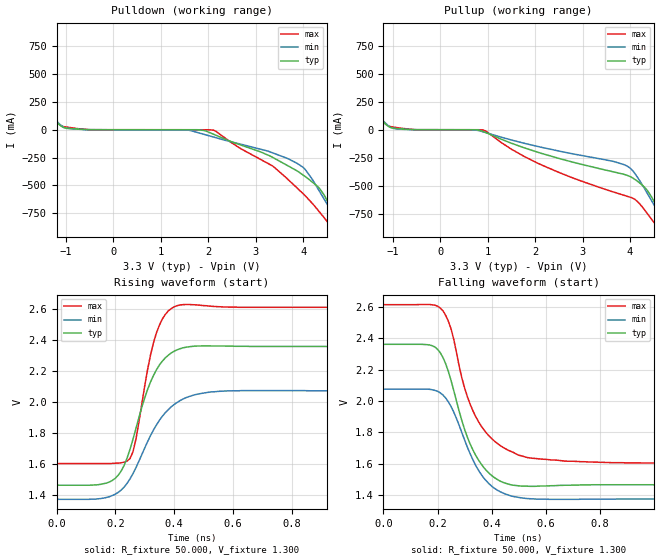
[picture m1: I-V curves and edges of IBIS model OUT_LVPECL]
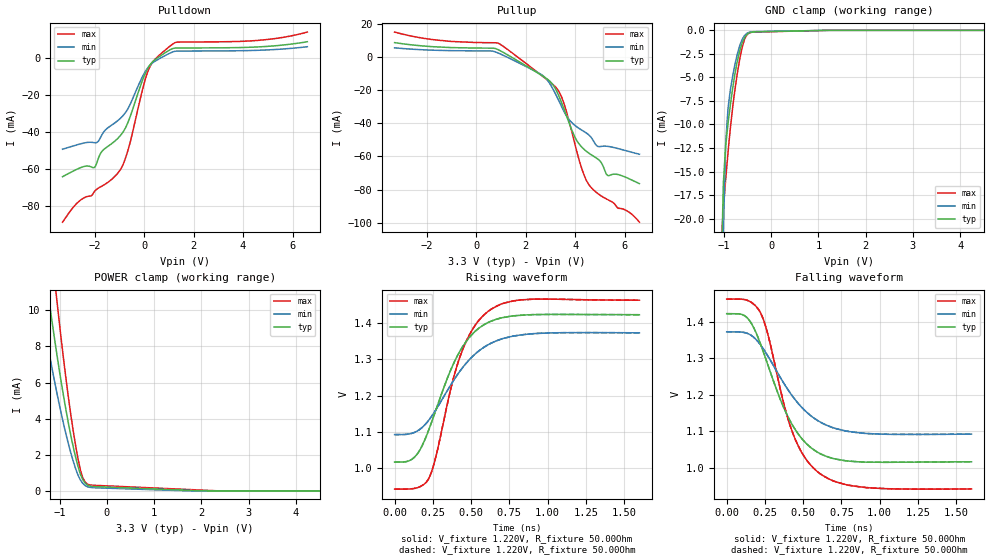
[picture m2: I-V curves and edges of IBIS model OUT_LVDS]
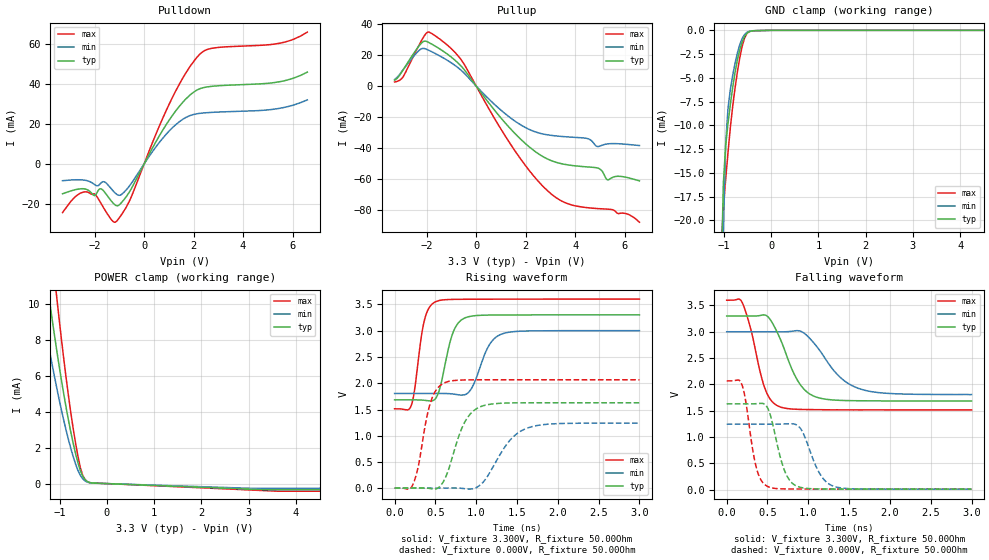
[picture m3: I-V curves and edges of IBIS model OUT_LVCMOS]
| Texas Instruments Incorporated
| Low-Noise Two-Channel 100-Mhz Clock Generator
| Marketing part#   Voltage Range   Package-type   #pins/pkg drawing
| CDCM9102   3.0V - 3.6V   QFN   32-pin
[IBIS ver]   4.0
[File name]   cdcm9102.ibs
[File Rev]   1.0
[Date]   02/xx/2012
[Source]   Texas Instruments Incorporated.
   Analog-eLab, HPA
   12500 TI Blvd
   Dallas, TX -75243
   For Support e-mail: elab_scm_ibis@list.ti.com
[Notes]   Revision History
   Rev 1.0: 02/xx/2012
   - Initial version of the model
   - Model based on simulations
[Disclaimer] This model is designed as an aid for customers of Texas Instruments.
 TI and its licensors and suppliers make no warranties, either expressed
 or implied, with respect to this  model, including the warranties of
 merchantability or fitness for a particular purpose.
 The model is provided solely on an "as is" basis. The entire risk as to
 its quality and performance is with the customer.
[Copyright] (C)Copyright 2012 Texas Instruments Incorporated.
   All rights reserved.
|   Component CDCM61001RHB
[Component]   CDCM9102
[Manufacturer]  Texas Instruments Incorporated
[Package]   |32-pin QFN RHB package + 1 mount pad
|   typ   min   max
R_pkg   0.0803   0.0465   0.1059
L_pkg   1.2961nH   0.9741nH   1.5599nH
C_pkg   0.1651pF   0.1340pF   0.2122pF
[Pin] signal_name  model_name   R_pin   L_pin   C_pin
1   VDD2   POWER   0.00347   0.14167nH   1.00649pF
2   OUT1N   OUT   0.10591   1.55991nH   0.16987pF
3   OUT1P   OUT   0.09554   1.38887nH   0.1537pF
4   VDD1   POWER   0.04649   0.97408nH   0.19897pF
5   OUT0N   OUT   0.0911   1.31619nH   0.14955pF
6   OUT0P   OUT   0.09304   1.34796nH   0.15105pF
7   OE   INPUT   0.09755   1.42251nH   0.15426pF
8   NC   NC   0.00035   0.05145nH   0.04372pF
9   VDD3   POWER   0.05784   1.4044nH   0.19557pF
10   OS1   INPUT   0.10035   1.46771nH   0.16304pF
11   OS0   INPUT   0.0874   1.25397nH   0.14393pF
12   RESETB   INPUT   0.07979   1.12929nH   0.13396pF
13   NC   NC   0.07954   1.12339nH   0.13334pF
14   GND   GND   0.08671   1.23786nH   0.13819pF
15   NC   NC   0.00035   0.04801nH   0.05605pF
16   VDD4   POWER   0.05695   1.35534nH   0.18238pF
17   REGCAP2   NC   0.1063   1.56176nH   0.15246pF
18   VDD5   POWER   0.05405   1.20242nH   0.21216pF
19   REGCAP1   NC   0.09847   1.42827nH   0.15881pF
20   VDD6   POWER   0.04904   1.04789nH   0.20348pF
21   XIN   NC   0.09225   1.32579nH   0.14835pF
22   GND   GND   0.09116   1.30806nH   0.14707pF
23   OSCOUT   OSC_OUT_25M   0.0919   1.32091nH   0.14396pF
24   NC   NC   0.00035   0.05145nH   0.04372pF
25   NC   NC   0.00035   0.05146nH   0.04372pF
26   NC   NC   0.00035   0.04801nH   0.05605pF
27   NC   NC   0.00035   0.04727nH   0.05608pF
28   NC   NC   0.00035   0.04709nH   0.05608pF
29   NC   NC   0.00035   0.04709nH   0.05608pF
30   NC   NC   0.00035   0.04726nH   0.05609pF
31   NC   NC   0.00035   0.04801nH   0.05605pF
32   NC   NC   0.00035   0.05145nH   0.04372pF
[Diff_Pin]  inv_pin  vdiff   tdelay_typ  tdelay_min  tdelay_max
| Driver Pins   |  Rload = 50 OHM to VCC-2 termination
|   Vdiff_lvpecl = 0.915V and Vdiff_lvds=0.350V
3   2   NA   0ns   0ns   0ns
6   5   NA   0ns   0ns   0ns
[Model Selector]   OUT
OUT_LVCMOS   LVCMOS OUTPUT
OUT_LVDS   LVDS   OUTPUT
OUT_LVPECL   LVPECL OUTPUT
| Models and submodels in the file (5): OUT_LVPECL (Output_ECL), OUT_LVDS (3-state), OUT_LVCMOS (3-state), OSC_OUT_25M (Output), INPUT (Input)
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|   OUT_LVPECL valid upto clock speed of 625MHz
[Model]   OUT_LVPECL
Model_type   Output_ECL
Cref = 0.0pF   |Timing specification test load capacitance value
Rref = 50.00Ohm
| variable   typ   min   max
|   Nominal PVT   Strong PVT   Weak PVT
C_comp   1.1664pF   1.1619pF   1.1764pF
[Model Spec]
Vref   1.3V   1.0V   1.6V
Vmeas   1.3V   1.0V   1.6V
[pullup reference]   3.3V   3.0V   3.6V
[pulldown reference]   3.3V   3.0V   3.6V
[GND clamp reference]   0V   0V   0V
| Junction Temperature (Ambient temp is 25C typ, 85C min,  -40C max)
[Temperature Range]   40.0   100.0   -40.0
[Voltage range]   3.3V   3.0V   3.6V
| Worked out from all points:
|   falling waveform, R_fixture 50.000, V_fixture 1.300: 20-80 % time 103ps typ, 110ps min, 118ps max; typ from 2.36 V to 1.47 V
|   rising waveform, R_fixture 50.000, V_fixture 1.300: 20-80 % time 91.4ps typ, 118ps min, 59.9ps max; typ from 1.47 V to 2.36 V
[Pulldown]
|   Voltage   I(typ)   I(min)   I(max)
-3.3V     1.332A     1.268A     1.424A
-2.68V    935.4mA    899.2mA    1.004A
-1.288V   115mA      119.3mA    116.2mA
-1.042V   18.84mA    20.53mA    27.56mA
1.586V    -109.5uA   -4.153mA   -17.03uA
2.111V    -40.58mA   -65.67mA   -4.131mA
3.352V    -247mA     -206.9mA   -324.1mA
3.992V    -405.1mA   -335.5mA   -571.5mA
4.342V    -525.1mA   -551.5mA   -737.5mA
4.689V    -781.1mA   -805.6mA   -932mA
4.89V     -953.1mA   -957.8mA   -1.114A
6.6V      -2.418A    -2.277A    -2.862A
[Pullup]
|   Voltage   I(typ)   I(min)   I(max)
-3.3V     1.332A     1.269A     1.435A
-2.63V    904.6mA    868.5mA    966.5mA
-1.29V    115.3mA    120.4mA    117.6mA
-1.067V   23.18mA    26.86mA    29.91mA
918mV     -17.48mA   -20.67mA   -4.542mA
2.059V    -201.7mA   -150.1mA   -300mA
3.672V    -378.5mA   -285.8mA   -559.7mA
4.02V     -422.7mA   -350mA     -605.8mA
4.317V    -519.2mA   -535mA     -722.3mA
4.665V    -763.2mA   -788.8mA   -915mA
4.838V    -904.1mA   -917.4mA   -1.054A
6.6V      -2.409A    -2.271A    -2.848A
[Ramp]
R_load = 50
|   typ   min   max
dV/dt_r   0.557474/9.12219e-11   0.420554/1.18318e-10   0.605849/5.99991e-11
dV/dt_f   0.557443/1.02721e-10   0.420514/1.10073e-10   0.605859/1.1832e-10
[Falling Waveform]
R_fixture = 50.000
V_fixture = 1.300
V_fixture_min = 1.000
V_fixture_max = 1.600
C_fixture = 0.000
|  time   V(typ)   V(min)   V(max)
0s        2.361V     2.075V     2.614V
170ps     2.357V     2.074V     2.615V
220ps     2.276V     2.037V     2.574V
250ps     2.128V     1.963V     2.457V
300ps     1.816V     1.749V     2.08V
340ps     1.654V     1.59V      1.902V
410ps     1.51V      1.442V     1.743V
500ps     1.458V     1.384V     NA
840ps     1.465V     1.373V     1.606V
1.7ns     1.465V     1.374V     1.605V
[Rising Waveform]
R_fixture = 50.000
V_fixture = 1.300
V_fixture_min = 1.000
V_fixture_max = 1.600
C_fixture = 0.000
|  time   V(typ)   V(min)   V(max)
0s        1.465V     1.374V     1.605V
180ps     1.486V     1.391V     1.605V
220ps     1.557V     1.434V     1.61V
250ps     1.696V     1.506V     1.637V
270ps     1.83V      1.577V     1.76V
310ps     2.084V     1.747V     2.213V
340ps     2.21V      1.854V     2.449V
410ps     2.339V     1.999V     2.624V
580ps     2.363V     2.074V     2.616V
1.7ns     2.361V     2.075V     2.614V
|   OUT_LVDS  valid upto clock speed of 625MHz
[Model]   OUT_LVDS
Model_type   3-state
Cref = 0.0pF   |Timing specification test load capacitance value
Rref = 50.00Ohm
| variable   typ   min   max
|   Nominal PVT   Strong PVT   Weak PVT
C_comp   1.1664pF   1.1619pF   1.1764pF
[Model Spec]
Vref   1.25V   1.15V   1.375V
Vmeas   1.25V   1.15V   1.375V
| Junction Temperature (Ambient temp is 25C typ, 85C min,  -40C max)
[Temperature Range]   40.0   100.0   -40.0
[Voltage range]   3.3V   3.0V   3.6V
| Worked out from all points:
|   slope of the pulldown table from 0 to 0.495 V, typ, clamps not added: 52.5 ohm
|   slope of the pullup table from 0 to 0.495 V, typ, clamps not added: 10.8 kohm
|   GND clamp passes 1 mA (typ) near -0.58 V on its own axis
|   POWER clamp passes 1 mA (typ) near -0.57 V on its own axis
|   falling waveform, V_fixture 1.220V, R_fixture 50.00Ohm: 20-80 % time 240ps typ, 280ps min, 211ps max; typ from 1.42 V to 1.02 V
|   rising waveform, V_fixture 1.220V, R_fixture 50.00Ohm: 20-80 % time 239ps typ, 282ps min, 200ps max; typ from 1.02 V to 1.42 V
|   rising waveform, V_fixture 1.220V, R_fixture 50.00Ohm: 20-80 % time 239ps typ, 282ps min, 200ps max; typ from 1.02 V to 1.42 V
|   falling waveform, V_fixture 1.220V, R_fixture 50.00Ohm: 20-80 % time 240ps typ, 280ps min, 211ps max; typ from 1.42 V to 1.02 V
[Pulldown]
|   Voltage   I(typ)   I(min)   I(max)
-3.3V     -64.32mA   -49.44mA   -88.92mA
-2.703V   -60.19mA   -47.03mA   -78.49mA
-2.007V   -59.31mA   -45.92mA   -72.26mA
-1.708V   -50.67mA   -41.67mA   -69.4mA
-961.8mV  -42.07mA   -32.76mA   -60.51mA
-613.6mV  -33.57mA   -26.49mA   -48.17mA
-66.33mV  -12.2mA    -10.21mA   -17.29mA
182.4mV   -4.943mA   -4.832mA   -6.331mA
431.2mV   -1.132mA   -1.934mA   -901.9uA
1.078V    4.53mA     2.728mA    6.643mA
4.909V    6.12mA     4.227mA    9.792mA
6.6V      8.704mA    6.006mA    13.92mA
[GND Clamp]
|   Voltage   I(typ)   I(min)   I(max)
-3.3V     -4.022A    -3.907A    -4.266A
-1.061V   -27.23mA   -43.89mA   -23.06mA
-1.012V   -16.24mA   -21.24mA   -18.95mA
-961.8mV  -12.25mA   -11.96mA   -15.82mA
-912.1mV  -9.874mA   -8.274mA   -12.94mA
-862.3mV  -7.89mA    -6.288mA   -10.34mA
-762.8mV  -4.522mA   -3.552mA   -6.176mA
-663.3mV  -2.151mA   -1.601mA   -3.015mA
-563.8mV  -779.3uA   -554.1uA   -972.9uA
-464.3mV  -264.9uA   -209.2uA   -276uA
1.227V    0A         -449.7nA   0A
6.6V      0A         0A         0A
[Pullup]
|   Voltage   I(typ)   I(min)   I(max)
-3.3V     8.704mA    5.566mA    15.07mA
878.9mV   4.518mA    2.501mA    8.413mA
2.521V    -9.902mA   -9.588mA   -9.69mA
3.068V    -16.07mA   -18.35mA   -16.17mA
3.416V    -26.18mA   -28.72mA   -22.91mA
4.013V    -48.96mA   -41.51mA   -53.82mA
4.312V    -55.01mA   -44.53mA   -69.18mA
4.56V     -58.06mA   -47.08mA   -77.11mA
4.909V    -61.49mA   -53.91mA   -82.32mA
5.307V    -71.46mA   -53.89mA   -85.99mA
5.754V    -71.01mA   -55.33mA   -91.31mA
6.6V      -76.42mA   -58.67mA   -99.7mA
[POWER Clamp]
|   Voltage   I(typ)   I(min)   I(max)
-3.3V     434.9mA    385mA      510.3mA
-1.459V   15.25mA    11.2mA     21.25mA
-1.41V    14.21mA    10.41mA    19.82mA
-1.26V    11.23mA    8.169mA    15.68mA
-1.211V   10.27mA    7.457mA    14.36mA
-1.061V   7.576mA    5.441mA    10.58mA
-862.3mV  4.403mA    3.086mA    6.102mA
-663.3mV  1.864mA    1.229mA    2.504mA
-514.1mV  630uA      424.6uA    736.8uA
-414.6mV  324.6uA    230.2uA    378.2uA
2.371V    0A         0A         2.594uA
6.6V      0A         0A         0A
[Ramp]
R_load = 50.00Ohm
|   typ   min   max
dV/dt_r   243.237mV/238.776ps 168.023mV/281.936ps 311.885mV/199.972ps
dV/dt_f   243.237mV/239.793ps 168.023mV/279.558ps 311.885mV/211.102ps
[Falling Waveform]
V_fixture = 1.220V
V_fixture_min = 1.232V
V_fixture_max = 1.200V
R_fixture = 50.00Ohm
|   Time   V(typ)   V(min)   V(max)
0s        1.422V     1.373V     1.462V
130ps     1.413V     1.369V     1.46V
220ps     1.34V      1.338V     1.425V
266ps     1.286V     1.308V     1.371V
372ps     1.166V     1.233V     1.178V
428ps     1.119V     1.198V     1.1V
503ps     1.074V     1.16V      1.034V
603ps     1.041V     1.128V     986.5mV
897ps     1.016V     1.095V     946.9mV
1.6ns     1.017V     1.092V     942.4mV
[Rising Waveform]
V_fixture = 1.220V
V_fixture_min = 1.232V
V_fixture_max = 1.200V
R_fixture = 50.00Ohm
|   Time   V(typ)   V(min)   V(max)
0s        1.017V     1.092V     942.4mV
128ps     1.03V      1.098V     944.3mV
223ps     1.105V     1.132V     971.5mV
265ps     1.154V     1.158V     1.024V
370ps     1.274V     1.231V     1.223V
429ps     1.324V     1.268V     1.309V
508ps     1.369V     1.307V     1.381V
610ps     1.401V     1.339V     1.431V
826ps     1.421V     1.367V     1.463V
1.6ns     1.422V     1.373V     1.462V
[Rising Waveform]
V_fixture = 1.220V
V_fixture_min = 1.232V
V_fixture_max = 1.200V
R_fixture = 50.00Ohm
|   Time   V(typ)   V(min)   V(max)
0s        1.017V     1.092V     942.4mV
128ps     1.03V      1.098V     944.3mV
223ps     1.105V     1.132V     971.5mV
265ps     1.154V     1.158V     1.024V
370ps     1.274V     1.231V     1.223V
429ps     1.324V     1.268V     1.309V
508ps     1.369V     1.307V     1.381V
610ps     1.401V     1.339V     1.431V
826ps     1.421V     1.367V     1.463V
1.6ns     1.422V     1.373V     1.462V
[Falling Waveform]
V_fixture = 1.220V
V_fixture_min = 1.232V
V_fixture_max = 1.200V
R_fixture = 50.00Ohm
|   Time   V(typ)   V(min)   V(max)
0s        1.422V     1.373V     1.462V
130ps     1.413V     1.369V     1.46V
220ps     1.34V      1.338V     1.425V
266ps     1.286V     1.308V     1.371V
372ps     1.166V     1.233V     1.178V
428ps     1.119V     1.198V     1.1V
503ps     1.074V     1.16V      1.034V
603ps     1.041V     1.128V     986.5mV
897ps     1.016V     1.095V     946.9mV
1.6ns     1.017V     1.092V     942.4mV
|   OUT_LVCMOS valid upto clock speed of 125MHz
[Model]   OUT_LVCMOS
Model_type   3-state
Cref = 5pF   |Timing specification test load capacitance value
Rref = 22Ohm
| variable   typ   min   max
|   Nominal PVT   Strong PVT   Weak PVT
C_comp   1.1795pF   1.1753pF   1.1905pF
[Model Spec]
|Timing spec test load voltage corners 0.45*VCC
Vmeas   3.3V   3.0V   3.6V
Vref   3.3V   3.0V   3.6V
| Junction Temperature (Ambient temp is 15C typ, 85C min,  -40C max)
[Temperature Range]   40.0   100.0   -40.0
[Voltage range]   3.3V   3.0V   3.6V
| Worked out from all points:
|   slope of the pulldown table from 0 to 0.495 V, typ, clamps not added: 43.1 ohm
|   slope of the pullup table from 0 to 0.495 V, typ, clamps not added: 46.8 ohm
|   GND clamp passes 1 mA (typ) near -0.59 V on its own axis
|   POWER clamp passes 1 mA (typ) near -0.60 V on its own axis
|   falling waveform, V_fixture 3.300V, R_fixture 50.00Ohm: 20-80 % time 273ps typ, 381ps min, 195ps max; typ from 3.3 V to 1.68 V
|   rising waveform, V_fixture 3.300V, R_fixture 50.00Ohm: 20-80 % time 148ps typ, 187ps min, 113ps max; typ from 1.68 V to 3.3 V
|   rising waveform, V_fixture 0.000V, R_fixture 50.00Ohm: 20-80 % time 221ps typ, 316ps min, 155ps max; typ from 0.008 V to 1.63 V
|   falling waveform, V_fixture 0.000V, R_fixture 50.00Ohm: 20-80 % time 162ps typ, 202ps min, 127ps max; typ from 1.63 V to 0.008 V
[Pulldown]
|   Voltage   I(typ)   I(min)   I(max)
-3.3V     -14.95mA   -8.415mA   -24.39mA
-2.753V   -12.82mA   -7.935mA   -16.11mA
-2.305V   -12.89mA   -8.403mA   -14.07mA
-2.007V   -15.89mA   -10.33mA   -15.03mA
-1.708V   -12.72mA   -9.15mA    -20.53mA
-1.31V    -18.83mA   -12.71mA   -28.14mA
-1.111V   -20.97mA   -15.21mA   -28.7mA
-613.6mV  -14.42mA   -11.37mA   -19.11mA
1.227V    25.73mA    19.09mA    35.34mA
2.371V    38.15mA    25.5mA     56.21mA
5.506V    41.26mA    27.93mA    60.55mA
6.6V      46.01mA    32.09mA    66.07mA
[GND Clamp]
|   Voltage   I(typ)   I(min)   I(max)
-3.3V     -4.022A    -3.907A    -4.266A
-1.061V   -27.1mA    -43.78mA   -22.92mA
-1.012V   -16.12mA   -21.13mA   -18.81mA
-961.8mV  -12.12mA   -11.85mA   -15.68mA
-912.1mV  -9.749mA   -8.168mA   -12.8mA
-862.3mV  -7.765mA   -6.182mA   -10.2mA
-762.8mV  -4.397mA   -3.446mA   -6.035mA
-663.3mV  -2.026mA   -1.495mA   -2.874mA
-613.6mV  -1.222mA   -859.7uA   -1.685mA
-563.8mV  -654uA     -448.1uA   -831.8uA
-464.3mV  -139.6uA   -103.1uA   -134.9uA
6.6V      0A         0A         0A
[Pullup]
|   Voltage   I(typ)   I(min)   I(max)
-3.3V     3.837mA    4.269mA    2.648mA
-2.952V   10.6mA     10.65mA    6.074mA
-2.206V   27.94mA    24.19mA    29.64mA
-1.808V   27.26mA    22.3mA     34.1mA
-613.6mV  12.99mA    10.29mA    17.12mA
1.476V    -29.18mA   -21.64mA   -39.75mA
2.869V    -47.09mA   -31.51mA   -67.51mA
3.764V    -51.15mA   -32.97mA   -76.49mA
4.56V     -52.39mA   -34.3mA    -78.83mA
4.958V    -53.3mA    -39.09mA   -79.33mA
5.307V    -60.7mA    -37.42mA   -79.64mA
6.6V      -61.35mA   -38.48mA   -88.1mA
[POWER Clamp]
|   Voltage   I(typ)   I(min)   I(max)
-3.3V     434.6mA    384.9mA    510mA
-1.41V    14mA       10.26mA    19.54mA
-1.26V    11.01mA    8.017mA    15.4mA
-1.211V   10.06mA    7.305mA    14.08mA
-1.061V   7.362mA    5.289mA    10.3mA
-862.3mV  4.189mA    2.934mA    5.822mA
-663.3mV  1.65mA     1.077mA    2.224mA
-563.8mV  716.6uA    457.4uA    895uA
-514.1mV  416uA      272.5uA    457uA
-414.6mV  110.6uA    78.08uA    98.41uA
3.615V    -340.9uA   -259.7uA   -422.6uA
6.6V      -340.9uA   -259.7uA   -422.6uA
[Ramp]
R_load = 50.00Ohm
|   typ   min   max
dV/dt_r   972.593mV/220.451ps 741.202mV/315.379ps   1.235V/154.381ps
dV/dt_f   969.834mV/273.026ps 716.631mV/380.535ps   1.252V/194.850ps
[Falling Waveform]
V_fixture = 3.300V
V_fixture_min = 3.000V
V_fixture_max = 3.600V
R_fixture = 50.00Ohm
|   Time   V(typ)   V(min)   V(max)
0s        3.3V       3V         3.6V
192ps     3.3V       3V         3.549V
294ps     3.299V     3V         3.057V
462ps     3.32V      3V         1.952V
630ps     2.954V     2.999V     1.587V
870ps     2.07V      3.021V     1.525V
1.09ns    1.762V     2.745V     1.519V
1.363ns   1.697V     2.176V     1.515V
1.61ns    1.688V     1.925V     1.513V
3ns       1.684V     1.806V     1.514V
[Rising Waveform]
V_fixture = 3.300V
V_fixture_min = 3.000V
V_fixture_max = 3.600V
R_fixture = 50.00Ohm
|   Time   V(typ)   V(min)   V(max)
0s        1.684V     1.806V     1.514V
203ps     1.684V     1.806V     1.573V
361ps     1.677V     1.806V     3.17V
502ps     1.709V     1.806V     3.549V
714ps     2.955V     1.795V     3.594V
866ps     3.244V     1.785V     3.596V
968ps     3.281V     1.977V     3.597V
1.164ns   3.296V     2.738V     3.598V
1.318ns   3.298V     2.939V     3.598V
3ns       3.3V       3V         3.6V
[Rising Waveform]
V_fixture = 0.000V
V_fixture_min = 0.000V
V_fixture_max = 0.000V
R_fixture = 50.00Ohm
|   Time   V(typ)   V(min)   V(max)
0s        7.63mV     6.612mV    8mV
223ps     7.766mV    6.6mV      68.68mV
288ps     8.394mV    6.591mV    404mV
438ps     -1.772mV   6.581mV    1.623V
613ps     173.8mV    7.047mV    2.01V
857ps     1.253V     -4.356mV   2.062V
1.057ns   1.557V     76.18mV    2.065V
1.401ns   1.625V     893.1mV    2.065V
1.607ns   1.628V     1.136V     2.065V
3ns       1.629V     1.242V     2.066V
[Falling Waveform]
V_fixture = 0.000V
V_fixture_min = 0.000V
V_fixture_max = 0.000V
R_fixture = 50.00Ohm
|   Time   V(typ)   V(min)   V(max)
0s        1.629V     1.242V     2.066V
185ps     1.628V     1.242V     2V
229ps     1.628V     1.242V     1.72V
362ps     1.632V     1.242V     425.3mV
505ps     1.54V      1.242V     55.67mV
710ps     355.6mV    1.247V     11.33mV
861ps     63.5mV     1.225V     9.348mV
1.136ns   10.45mV    313.8mV    8.631mV
1.311ns   8.724mV    61.63mV    8.41mV
3ns       7.63mV     6.612mV    8mV
